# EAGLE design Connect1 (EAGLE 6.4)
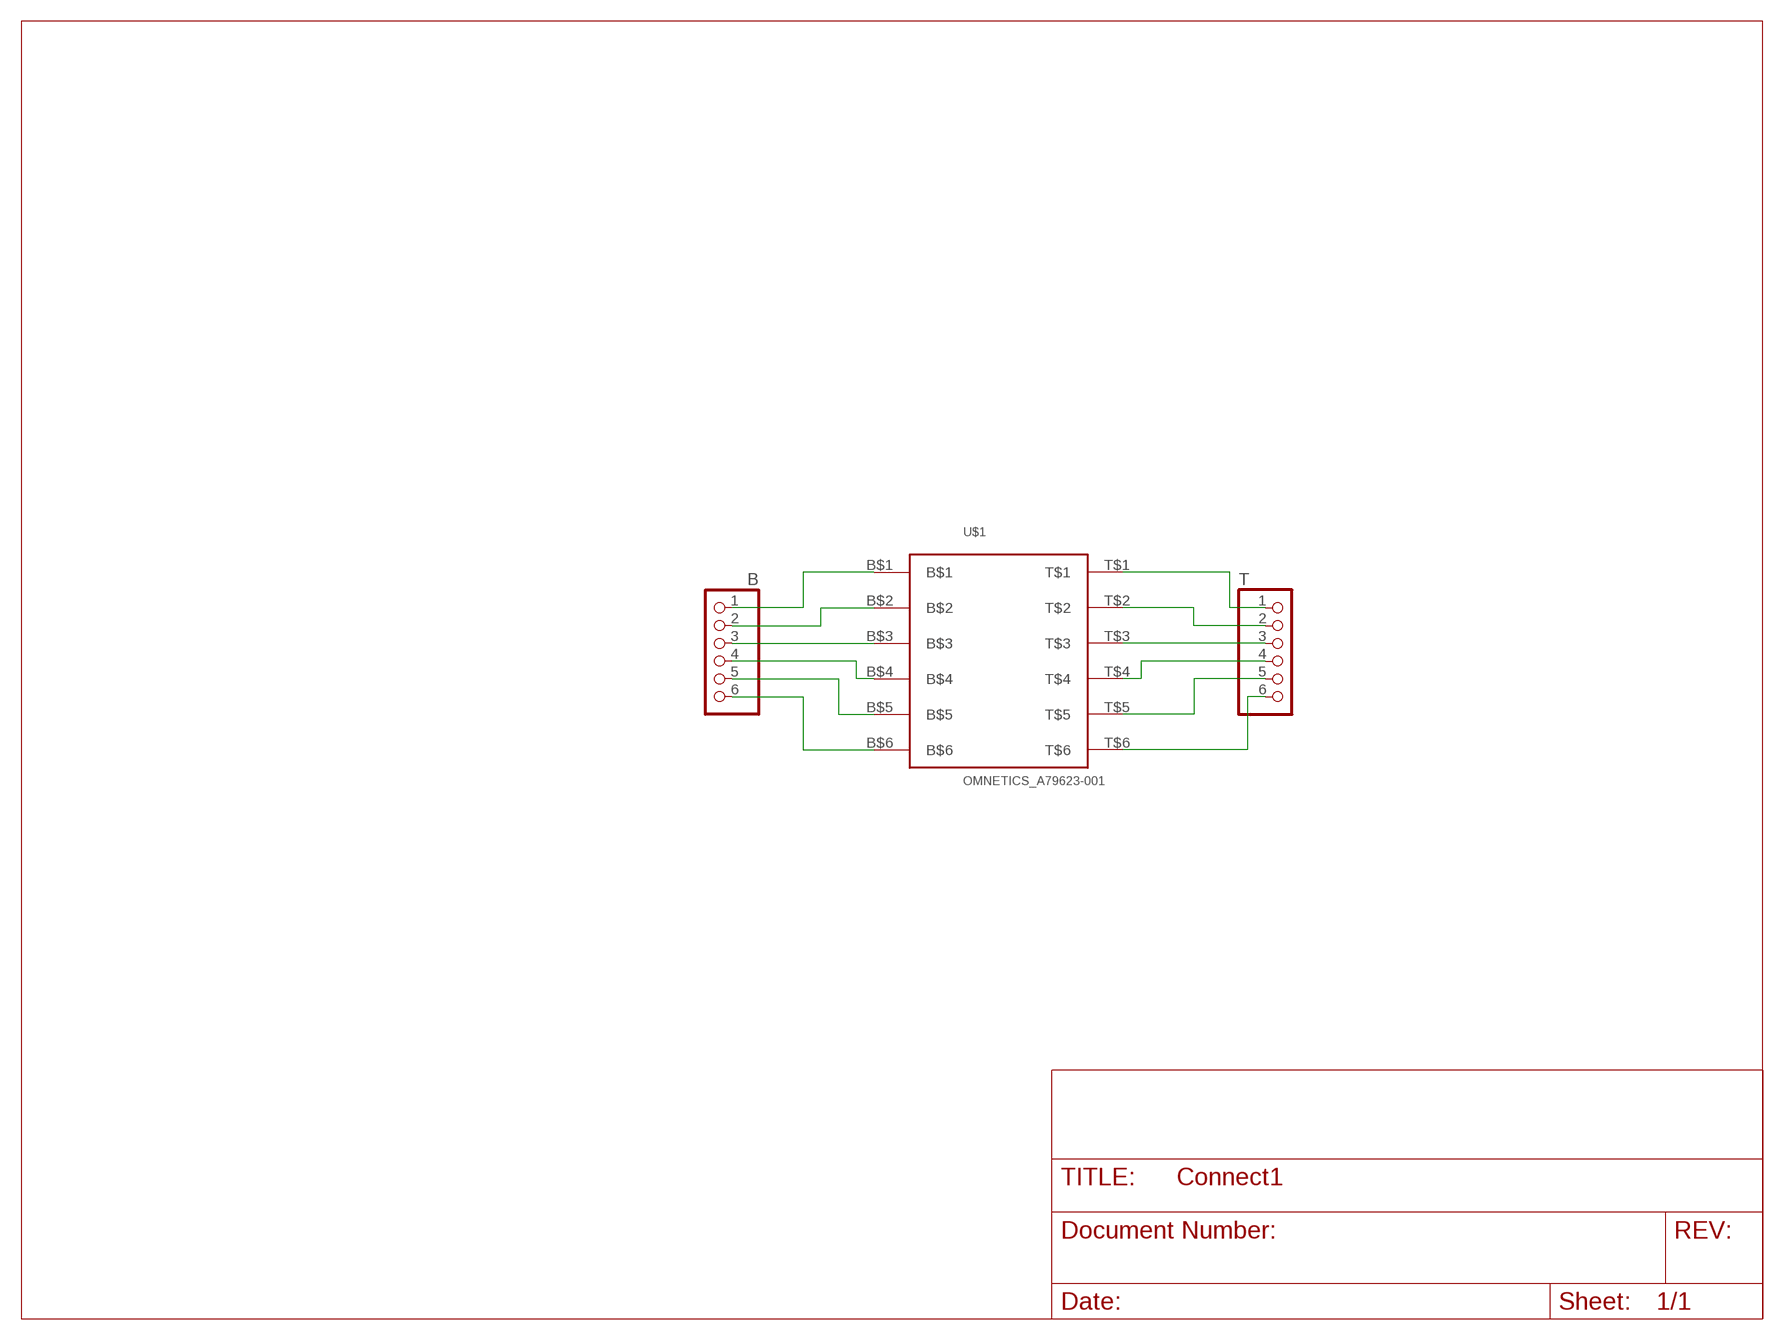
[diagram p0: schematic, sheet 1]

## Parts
B  PINHD-1X6  [1X06]
T  PINHD-1X6  [1X06]
U$1  OMNETICS_A79623-001  [OMNETICS_A79623-001]

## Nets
N$1: B.1 U$1.B$1
N$2: B.2 U$1.B$2
N$3: B.3 U$1.B$3
N$4: B.4 U$1.B$4
N$5: B.5 U$1.B$5
N$6: B.6 U$1.B$6
N$7: T.1 U$1.T$1
N$8: T.2 U$1.T$2
N$9: T.3 U$1.T$3
N$10: T.4 U$1.T$4
N$11: T.5 U$1.T$5
N$12: T.6 U$1.T$6

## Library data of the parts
B T = pinhead:PINHD-1X6: PIN HEADER
U$1 = omnetics_vic:OMNETICS_A79623-001

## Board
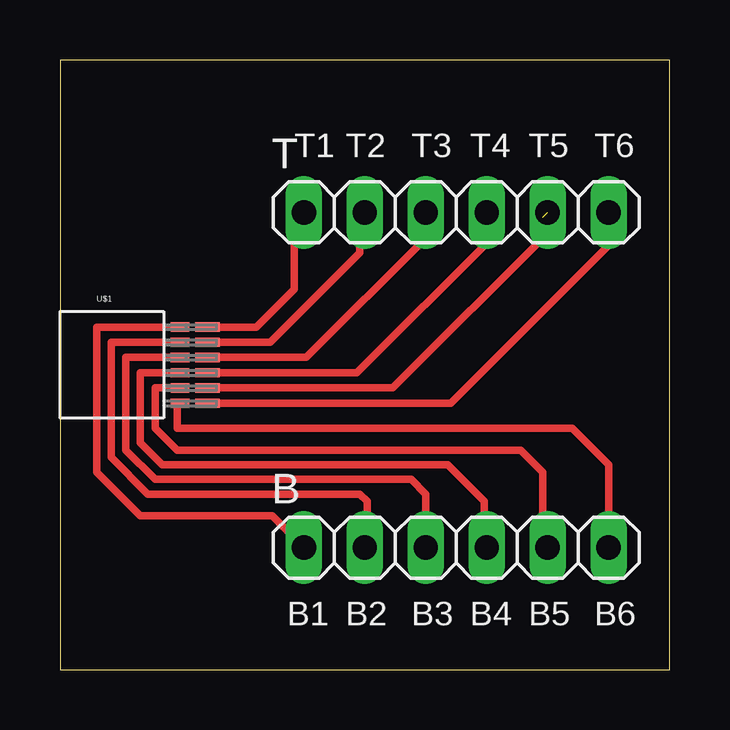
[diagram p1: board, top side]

Size 25.4 x 25.4 mm. Coordinates in mm from the lower left corner, seen from the top.
Outline: 0,0 25.4,0 25.4,25.4 0,25.4 0,0
Copper layers (1*16): Top 0.035mm / dielectric 1.5mm / Bottom 0.035mm
Design rules "default": minimum track width 10mil, minimum drill 24mil, track to track 8mil, track to pad 8mil, pad to pad 8mil, via to via 8mil, smd to smd 8mil, copper to edge 40mil, drill to drill 8mil, minimum pad ring 10mil, minimum via ring 8mil, stop-mask expansion 4mil, vias tented up to drill 0mil, thermal gap 10mil

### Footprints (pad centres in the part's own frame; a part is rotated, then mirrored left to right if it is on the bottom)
1X06 = drill 1.016 long: 1 -6.35,0; 2 -3.81,0; 3 -1.27,0; 4 1.27,0; 5 3.81,0; 6 6.35,0
OMNETICS_A79623-001 = smd 0.762 x 0.381: B$1 2.845,1.575; B$2 2.845,0.94; B$3 2.845,0.305; B$4 2.845,-0.33; B$5 2.845,-0.965; B$6 2.845,-1.6 | smd 1.016 x 0.381: T$1 3.988,1.575; T$2 3.988,0.94; T$3 3.988,0.305; T$4 3.988,-0.33; T$5 3.988,-0.965; T$6 3.988,-1.6

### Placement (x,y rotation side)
B  16.51,5.08 0 top
T  16.51,19.05 0 top
U$1  2.16,12.7 0 top

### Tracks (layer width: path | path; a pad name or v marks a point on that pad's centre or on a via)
N$1
  Top 0.305: U$1.B$1 1.52,14.28 1.52,8.23 3.35,6.4 8.84,6.4 B.1
N$2
  Top 0.305: U$1.B$2 2.13,13.64 2.13,8.84 3.66,7.32 12.5,7.32 12.8,7.01 12.8,5.18 B.2
N$3
  Top 0.305: U$1.B$3 2.74,13.01 2.74,9.14 3.96,7.92 14.63,7.92 15.24,7.32 B.3
N$4
  Top 0.305: U$1.B$4 3.35,12.37 3.35,9.45 4.27,8.53 16.15,8.53 17.68,7.01 17.68,5.18 B.4
N$5
  Top 0.305: U$1.B$5 3.96,11.73 3.96,10.06 4.88,9.14 19.2,9.14 20.12,8.23 20.12,5.28 B.5
N$6
  Top 0.305: U$1.B$6 4.88,11.1 4.88,10.06 21.34,10.06 22.86,8.53 B.6
N$7
  Top 0.305: U$1.T$1 8.18,14.28 9.75,15.85 9.75,18.64 T.1
N$8
  Top 0.305: U$1.T$2 8.76,13.64 12.5,17.37 12.5,18.85 T.2
N$9
  Top 0.305: U$1.T$3 10.26,13.01 15.24,17.98 T.3
N$10
  Top 0.305: U$1.T$4 12.37,12.37 17.98,17.98 17.98,18.85 T.4
N$11  (1 unrouted)
  Top 0.305: U$1.T$5 13.87,11.73 20.42,18.29 20.42,18.95 T.5
N$12
  Top 0.305: U$1.T$6 16.28,11.1 22.86,17.68 T.6

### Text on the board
tNames: T1 | T2 | T3 | T4 | T5 | T6 | B1 | B2 | B3 | B4 | B5 | B6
